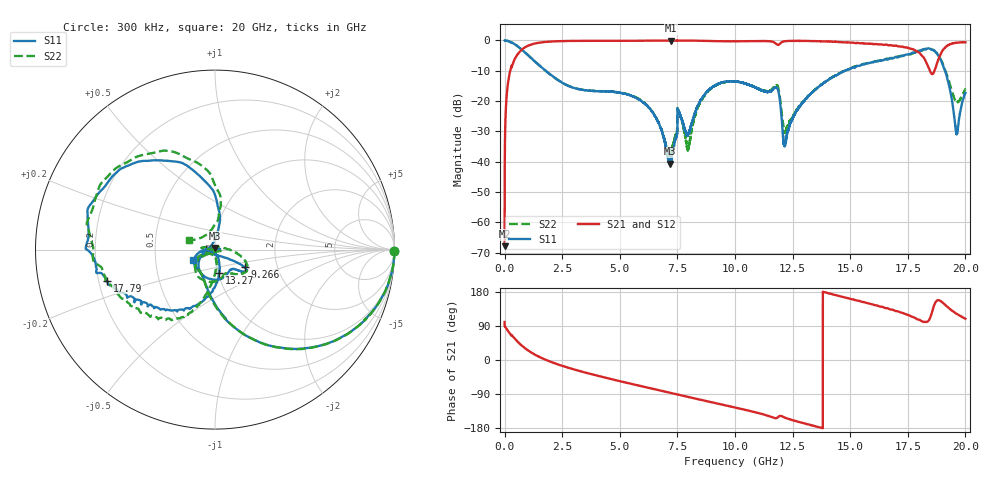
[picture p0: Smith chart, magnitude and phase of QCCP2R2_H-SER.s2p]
!{QCCP2R2}
!Johanson Technology Inc.
!www.johansontechnology.com
!Test Board Conditions:
!Substrate Type  RO4350B
!Substrate Thickness  20 mil
!Substrate Dk  3.66
!TL Type: GCPW
!TL Trace Width  36 mil
!TL Gap  12 mil
!Electrode orientation  Horizontal
!DUT TOPOLOGY	SERIES
!Mounting Pad LxW  26x36 mil
! Created Sat Jan  9 18:27:04 2021
# hz S ma R 50
! 2 Port Network Data from SP1.SP block
! freq  magS11  angS11  magS21  angS21  magS12  angS12  magS22  angS22
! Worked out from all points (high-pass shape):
!   20001 points, 300 kHz to 20 GHz, reference 50 ohm
!   highest |S21| = -0.03 dB at 7.228 GHz (marker M1); lowest = -67.8 dB at 300 kHz (marker M2)
!   |S21| within 3 dB of the highest: 748.6 MHz to 17.76 GHz (17.02 GHz wide, 184 % of centre); 19.03 GHz to end of sweep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
!   lowest |S11| = -40.6 dB at 7.192 GHz (marker M3), VSWR 1.02, Z = 50.2 + j0.916 ohm
!   |S11| at or under -10 dB: 1.782 GHz to 14.77 GHz (12.99 GHz wide, 157 % of centre); 14.77022 GHz to 14.7708 GHz (584.3 kHz wide, 0.00396 % of centre); 19.12 GHz to end of sweep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
!   |S22| runs from -38.1 to 0.0 dB; largest |S21 - S12| = 0.015
!   S11 on the Smith chart (normalised r, x): 300 kHz: open; 9.266 GHz: 1.37, -0.28; 13.27 GHz: 1.01, -0.27; 17.79 GHz: 0.23, -0.13; 20 GHz: 0.78, -0.09
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300000  0.9962 -0.3  0.0004057 100.3  0.0004386 92.2  0.9972 -0.4
1.313e8  0.9833 -11.5  0.1778 78.1  0.1778 78.2  0.9831 -11.6
4.813e8  0.8465 -36.1  0.5266 53.6  0.5268 53.6  0.8477 -36.2
1.4983e9  0.3891 -81.8  0.9188 8.2  0.9189 8.2  0.3913 -81.4
3.3343e9  0.1544 -120.5  0.9847 -30.4  0.9844 -30.4  0.1546 -119.6
6.6673e9  0.04509 173.6  0.994 -79.2  0.9942 -79.3  0.04517 -147.9
7.1923e9  0.009329 77.9  0.9951 -86.6  0.9944 -86.6  0.01336 -65.4
7.2283e9  0.0105 58.4  0.9968 -87.0  0.9949 -87.0  0.01428 -53.8
7.6003e9  0.06243 -163.6  0.9929 -92.4  0.9922 -92.3  0.06292 166.0
7.9693e9  0.02921 -90.8  0.9933 -97.5  0.993 -97.5  0.01601 76.5
9.2663e9  0.1931 -30.6  0.9725 -115.3  0.972 -115.3  0.1906 -23.0
1.00003e10  0.2099 -35.9  0.9689 -125.3  0.9703 -125.4  0.2106 -36.1
1.18033e10  0.1657 -98.2  0.8709 -153.2  0.8708 -153.2  0.1816 -106.7
1.21703e10  0.01871 -96.4  0.9715 -152.2  0.9719 -152.1  0.03096 -119.3
1.32743e10  0.1308 -79.5  0.9783 -171.4  0.9781 -171.5  0.1323 -89.7
1.33343e10  0.1376 -80.1  0.9755 -172.4  0.9761 -172.4  0.1373 -90.0
1.66673e10  0.4936 -143.5  0.8299 135.4  0.833 134.9  0.4978 -129.9
1.77913e10  0.6266 -164.0  0.6981 111.9  0.6913 111.9  0.6326 -163.9
1.83613e10  0.738 164.2  0.3876 101.5  0.3897 101.5  0.7212 159.0
1.88703e10  0.5292 112.5  0.5372 157.6  0.5362 157.1  0.5332 107.0
1.96153e10  0.02906 141.7  0.9206 122.0  0.9221 122.3  0.0955 117.4
2e10  0.1364 -154.1  0.9343 109.0  0.93 109.0  0.1565 160.9
